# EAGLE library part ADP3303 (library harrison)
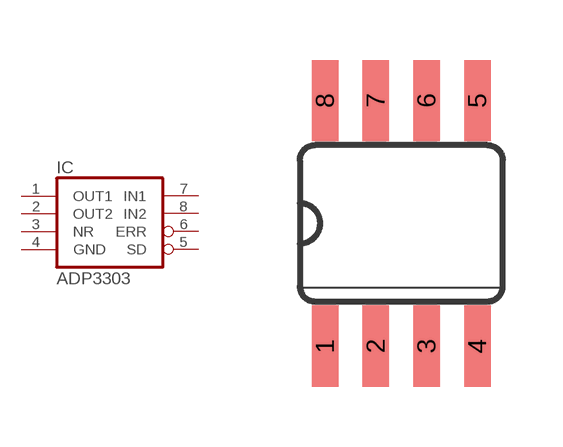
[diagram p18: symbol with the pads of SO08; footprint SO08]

Designator prefix IC

## ADP3303A  [SO08]
1  OUT1  pwr
2  OUT2  pwr
3  NR
4  GND  pwr
5  SD  in
6  ERR  out
7  IN1  pwr
8  IN2  pwr

## Footprint SO08 (pad centres in mm)
smd 0.66 x 2.032: 1 -1.905,-3.073; 2 -0.635,-3.073; 3 0.635,-3.073; 4 1.905,-3.073; 5 1.905,3.073; 6 0.635,3.073; 7 -0.635,3.073; 8 -1.905,3.073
